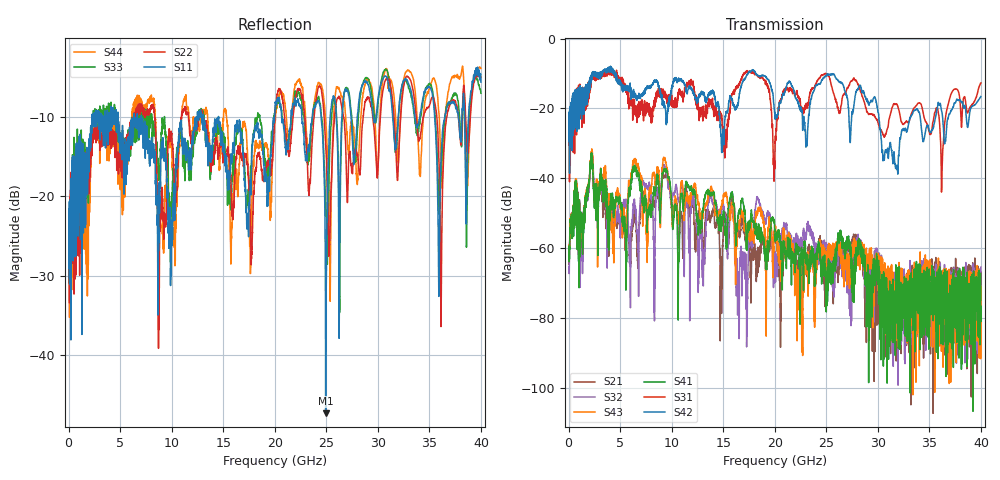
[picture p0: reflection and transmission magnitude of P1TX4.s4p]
!Agilent Technologies,N5245A,MY49151084,A.09.20.08
!Agilent N5245A: A.09.20.08
!Date: Thursday, March 01, 2012 14:18:31
!Correction: S11(Full 4 Port(1,2,3,4))
!S12(Full 4 Port(1,2,3,4))
!S13(Full 4 Port(1,2,3,4))
!S14(Full 4 Port(1,2,3,4))
!S21(Full 4 Port(1,2,3,4))
!S22(Full 4 Port(1,2,3,4))
!S23(Full 4 Port(1,2,3,4))
!S24(Full 4 Port(1,2,3,4))
!S31(Full 4 Port(1,2,3,4))
!S32(Full 4 Port(1,2,3,4))
!S33(Full 4 Port(1,2,3,4))
!S34(Full 4 Port(1,2,3,4))
!S41(Full 4 Port(1,2,3,4))
!S42(Full 4 Port(1,2,3,4))
!S43(Full 4 Port(1,2,3,4))
!S44(Full 4 Port(1,2,3,4))
!S4P File: Measurements: <S11,S12,S13,S14>,
!<S21,S22,S23,S24>,
!<S31,S32,S33,S34>,
!<S41,S42,S43,S44>:
# Hz S  dB  R 50
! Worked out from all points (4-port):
!   3996 points, 50 MHz to 40 GHz, reference 50 ohm
!   strongest paths, dB at 50 MHz, 10.04 GHz, 20.03 GHz, 30.02 GHz, 40 GHz:
!     S42: -23.5, -13.6, -22.2, -21.1, -16.6
!     S31: -26.5, -18.6, -29.5, -24.1, -12.7
!     S41: -59.4, -50.4, -55.9, -65.7, -81.0
!     S43: -59.1, -50.7, -54.9, -63.4, -71.0
!     S32: -65.3, -45.5, -62.4, -64.1, -65.5
!     S21: -61.1, -49.5, -57.4, -73.6, -71.8
!   lowest |S11| = -47.3 dB at 24.94 GHz (marker M1), VSWR 1.01, Z = 50.4 - j0.0997 ohm
!   |S11| at or under -10 dB: start of sweep to 2.262 GHz; 7.051 GHz to 12.46 GHz (5.408 GHz wide, 55.4 % of centre); 14.54 GHz to 19.98 GHz (5.438 GHz wide, 31.5 % of centre)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
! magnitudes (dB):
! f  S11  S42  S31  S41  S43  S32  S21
! 50 MHz  -24.5  -23.5  -26.5  -59.4  -59.1  -65.3  -61.1
! 2.2 GHz  -12.0  -10.5  -12.1  -35.5  -34.5  -34.8  -35.8
! 17.86 GHz  -12.9  -8.9  -9.7  -52.3  -56.6  -58.3  -62.0
! 19.99 GHz  -9.8  -21.4  -37.4  -55.0  -55.0  -62.4  -56.4
! 24.94 GHz  -47.3  -10.7  -10.0  -68.1  -62.4  -59.8  -69.6
! 31.79 GHz  -13.8  -36.7  -18.7  -78.1  -75.7  -70.1  -92.3
! 40 GHz  -5.6  -16.6  -12.7  -81.0  -71.0  -65.5  -71.8
